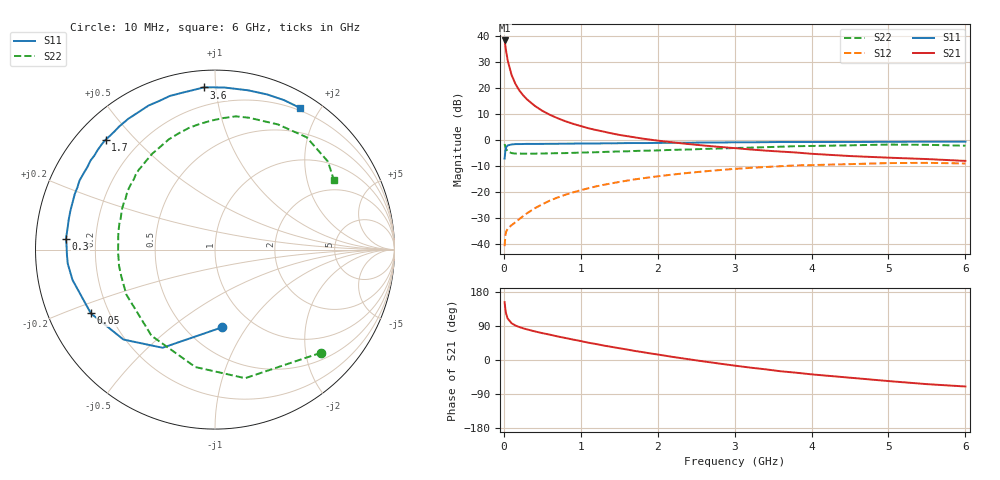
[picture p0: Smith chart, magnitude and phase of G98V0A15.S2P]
! SIEMENS Small Signal Semiconductors
! BFG235
! Si NPN RF Bipolar Junction Transistor in SOT223
! VCE = 8 V  IC = 150 mA
! Common Emitter S-Parameters:  July  1994
# GHz  S  MA  R  50
!  f  S11  S21  S12  S22
! GHz  MAG  ANG  MAG  ANG  MAG  ANG  MAG  ANG
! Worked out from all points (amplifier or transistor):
!   40 points, 10 MHz to 6 GHz, reference 50 ohm
!   highest |S21| = 38.2 dB at 10 MHz (marker M1)
!   |S21| within 3 dB of that: start of sweep to 24.56 MHz
!   unconditionally stable (mu >= 1): 459.2 MHz to 1.5 GHz
!   at 200 MHz: K = 0.80, MSG = 24.8 dB, |S12| = -30.5 dB
!   at 1.5 GHz: K = 1.00, MSG = 9.0 dB, |S12| = -16.2 dB
!   at 6 GHz: K = 0.88, MSG = 0.5 dB, |S12| = -9.1 dB
!   S11 on the Smith chart (normalised r, x): 10 MHz: 0.73, -0.78; 50 MHz: 0.13, -0.24; 300 MHz: 0.09, +0.04; 1.7 GHz: 0.09, +0.41; 3.6 GHz: 0.09, +0.93; 6 GHz: 0.17, +1.75
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0.01  0.4345 -84.6  80.93 152.6  0.009 63.5  0.824 -44.2
0.02  0.62 -118.1  63.96 133.8  0.0143 49.5  0.7359 -76.8
0.03  0.715 -135.5  50.23 121.9  0.0171 41.2  0.6634 -99.5
0.05  0.7775 -152.8  33.51 109.3  0.0194 33.9  0.5963 -126.4
0.1  0.8118 -168.0  17.7 97.1  0.0228 36.1  0.5539 -153.1
0.15  0.8242 -174.6  11.89 91.0  0.0259 42.7  0.5428 -164.3
0.2  0.8255 -178.0  8.907 87.1  0.0298 47.1  0.5423 -170.5
0.25  0.8271 178.7  7.174 83.7  0.034 51.1  0.5396 -174.8
0.3  0.8324 175.9  5.987 80.9  0.0385 53.8  0.5403 -178.4
0.4  0.8301 171.6  4.506 75.6  0.0479 56.6  0.5403 176.5
0.5  0.8323 168.0  3.597 70.9  0.0575 57.8  0.5442 172.3
0.6  0.8343 164.8  3.005 66.8  0.0678 57.8  0.548 168.4
0.8  0.8405 158.4  2.266 58.1  0.0878 56.3  0.5535 161.7
1.1  0.8464 149.4  1.661 45.6  0.1169 51.7  0.5712 152.7
1.4  0.852 142.2  1.325 34.6  0.1451 45.9  0.5893 144.5
1.7  0.864 134.9  1.112 24.0  0.1729 39.6  0.608 136.6
2.2  0.8744 123.6  0.889 8.0  0.2146 28.6  0.6389 123.1
3.2  0.8926 102.2  0.651 -20.0  0.2874 5.4  0.7044 97.3
3.6  0.9057 94.0  0.592 -29.8  0.3101 -4.4  0.7348 86.2
4.5  0.9064 78.3  0.486 -46.7  0.3397 -24.3  0.7806 63.3
5.5  0.9175 65.1  0.425 -63.7  0.3594 -46.3  0.798 38.0
6  0.9203 59.1  0.392 -69.9  0.3498 -54.7  0.7679 30.5
